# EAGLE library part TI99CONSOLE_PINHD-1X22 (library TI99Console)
PIN HEADER
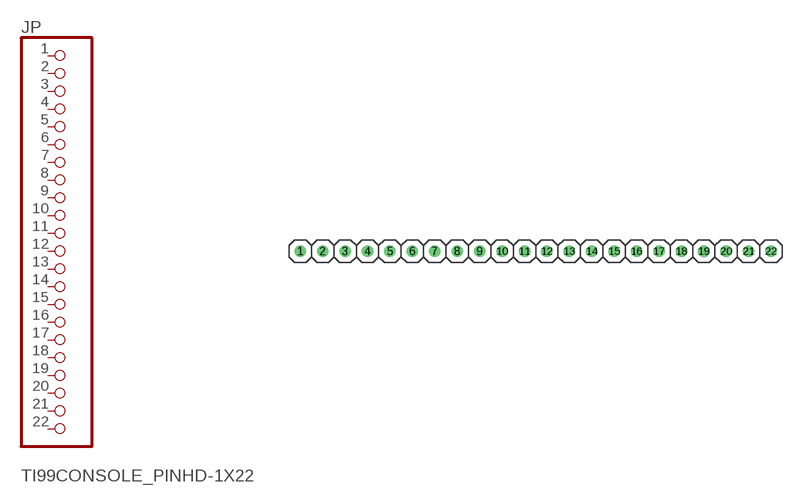
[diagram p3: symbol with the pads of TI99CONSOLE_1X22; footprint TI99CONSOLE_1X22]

Designator prefix JP

## TI99CONSOLE_PINHD-1X22  [TI99CONSOLE_1X22]
1  1  pas
2  2  pas
3  3  pas
4  4  pas
5  5  pas
6  6  pas
7  7  pas
8  8  pas
9  9  pas
10  10  pas
11  11  pas
12  12  pas
13  13  pas
14  14  pas
15  15  pas
16  16  pas
17  17  pas
18  18  pas
19  19  pas
20  20  pas
21  21  pas
22  22  pas

## Footprint TI99CONSOLE_1X22 (pad centres in mm)
PIN HEADER
drill 0.8: 1 -24.13,0; 2 -21.59,0; 3 -19.05,0; 4 -16.51,0; 5 -13.97,0; 6 -11.43,0; 7 -8.89,0; 8 -6.35,0; 9 -3.81,0; 10 -1.27,0; 11 1.27,0; 12 3.81,0; 13 6.35,0; 14 8.89,0; 15 11.43,0; 16 13.97,0; 17 16.51,0; 18 19.05,0; 19 21.59,0; 20 24.13,0; 21 26.67,0; 22 29.21,0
